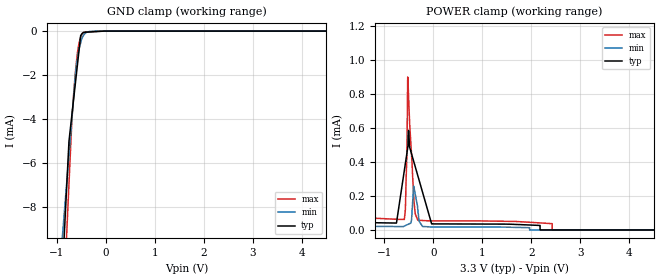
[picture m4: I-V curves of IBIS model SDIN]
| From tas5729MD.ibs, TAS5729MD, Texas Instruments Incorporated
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[Model]   SDIN
Model_type   Input
Vinl = .8
Vinh = 2
|   typ   min   max
C_comp   0.7443p   0.7440p   0.7473p
[Voltage Range]   3.3   3   3.6
[Temperature Range]   27   125   0
[Power Clamp Reference]   3.3   3   3.6
[GND Clamp Reference]   -0   -0   -0
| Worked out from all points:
|   GND clamp passes 1 mA (typ) near -0.56 V on its own axis
|   POWER clamp passes 1 mA (typ) near -3.27 V on its own axis
[GND Clamp]
|   Voltage   I(typ)   I(min)   I(max)
-3.3V     -1.514A    -1.357A    -1.56A
-1.01V    -16.37mA   -12.7mA    -19.44mA
-755.5mV  -5.027mA   -5.644mA   -6.97mA
-697.1mV  -3.847mA   -4.024mA   -4.108mA
-663.5mV  -3.171mA   -3.096mA   -2.981mA
-613.3mV  -2.157mA   -1.717mA   -1.618mA
-567.6mV  -1.236mA   -1.067mA   -777.7uA
-516.6mV  -207.7uA   -537.5uA   -275.9uA
-457mV    -57.17uA   -189.9uA   -86.11uA
-394mV    -48.76uA   -54.45uA   -36.92uA
-223.1mV  -25.94uA   -4.607uA   -18.85uA
6.6V      0A         0A         0A
[POWER Clamp]
|   Voltage   I(typ)   I(min)   I(max)
-3.3V     1.08mA     9.274mA    1.113mA
-2.875V   520.5uA    1.205mA    563.2uA
-2.536V   226.6uA    394.6uA    188.3uA
-1.687V   44.59uA    30.76uA    75.69uA
-755.5mV  40.68uA    20.26uA    62.9uA
-594.9mV  350uA      22.59uA    62.02uA
-544.3mV  447.4uA    29.43uA    425.3uA
-525.1mV  484.3uA    32.02uA    900uA
-400.3mV  400.7uA    255.7uA    179.6uA
-318.1mV  318.1uA    116.8uA    57.01uA
-37mV     35.73uA    17.83uA    53.38uA
6.6V      0A         0A         0A
